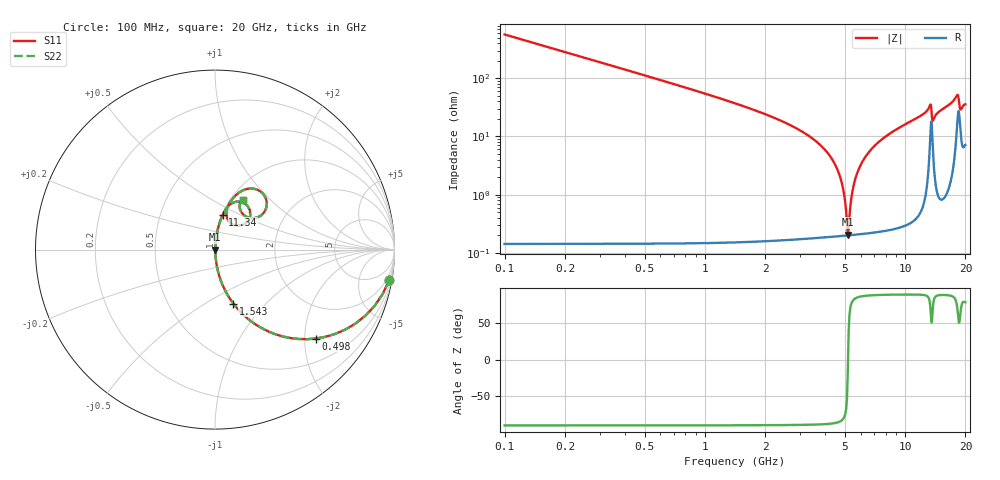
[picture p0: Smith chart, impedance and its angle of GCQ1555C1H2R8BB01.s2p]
!Murata Part Number: GCQ1555C1H2R8BB01
!These Parameters are Measured in Series Mode Connection
!Data Generated on Mar 13, 2026
!  o--ll--o
!Port1  Port2
!  o------o
!Operation Temp=25[degC], DC Bias Voltage=0[V]
!Freq. Start=100[MHz] Stop=20[GHz] 401[Steps]
# Hz S RI R 50
!Freq.(Hz) S11(Real) S11(Imag) S21(Real) S21(Imag) S12(Real) S12(Imag) S22(Real) S22(Imag)
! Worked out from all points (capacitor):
!   401 points, 100 MHz to 20 GHz, reference 50 ohm
!   read as one part in series: C = 2.8 pF near 199.5 MHz
!   lowest |Z| = 206 mohm at 5.175 GHz (marker M1)
!   series resonance near 5.187 GHz, so ESL is about 340 pH
!   S11 on the Smith chart (normalised r, x): 100 MHz: 1, -11; 498 MHz: 1.00, -2.26; 1.543 GHz: 1.00, -0.67; 11.34 GHz: 1.01, +0.41; 20 GHz: 1.14, +0.70
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1e8  0.9699 -0.1707  0.0301 0.1707  0.0301 0.1707  0.9699 -0.1707
2.99e8  0.782 -0.4125  0.218 0.4125  0.218 0.4125  0.782 -0.4125
4.98e8  0.5611 -0.4956  0.4389 0.4956  0.4389 0.4956  0.5611 -0.4956
9.4575e8  0.253 -0.4335  0.747 0.4335  0.747 0.4335  0.253 -0.4335
1.54275e9  0.1025 -0.3011  0.8975 0.3011  0.8975 0.3011  0.1025 -0.3011
3.43325e9  0.0103 -0.0921  0.9897 0.0921  0.9897 0.0921  0.0103 -0.0921
4.12975e9  0.00439 -0.0503  0.9956 0.0503  0.9956 0.0503  0.00439 -0.0503
4.62725e9  0.00255 -0.0251  0.9975 0.0251  0.9975 0.0251  0.00255 -0.0251
4.92575e9  0.00208 -0.0114  0.9979 0.0114  0.9979 0.0114  0.00208 -0.0114
5.1745e9  0.00198 -0.000541  0.998 0.000541  0.998 0.000541  0.00198 -0.000541
5.274e9  0.00201 0.00365  0.998 -0.00365  0.998 -0.00365  0.00201 0.00365
5.473e9  0.00216 0.0118  0.9978 -0.0118  0.9978 -0.0118  0.00216 0.0118
5.72175e9  0.00252 0.0216  0.9975 -0.0216  0.9975 -0.0216  0.00252 0.0216
6.7665e9  0.00572 0.0593  0.9943 -0.0593  0.9943 -0.0593  0.00572 0.0593
1.005e10  0.0286 0.1578  0.9714 -0.1578  0.9714 -0.1578  0.0286 0.1578
1.13435e10  0.0434 0.1945  0.9566 -0.1945  0.9566 -0.1945  0.0434 0.1945
1.338325e10  0.1803 0.2448  0.8197 -0.2448  0.8197 -0.2448  0.1803 0.2448
1.37315e10  0.0881 0.1478  0.9119 -0.1478  0.9119 -0.1478  0.0881 0.1478
1.67165e10  0.1242 0.31  0.8758 -0.31  0.8758 -0.31  0.1242 0.31
1.835825e10  0.2886 0.2605  0.7114 -0.2605  0.7114 -0.2605  0.2886 0.2605
1.885575e10  0.1651 0.1895  0.8349 -0.1895  0.8349 -0.1895  0.1651 0.1895
2e10  0.1572 0.2761  0.8428 -0.2761  0.8428 -0.2761  0.1572 0.2761
